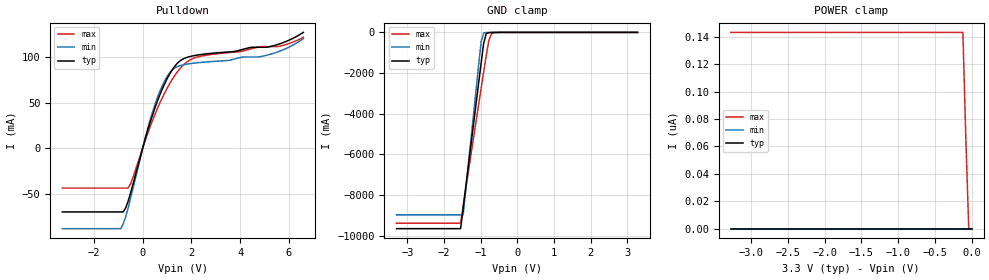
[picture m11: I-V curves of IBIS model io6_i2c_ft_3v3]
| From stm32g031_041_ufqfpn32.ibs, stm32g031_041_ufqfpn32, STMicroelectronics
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|   Model io6_i2c_ft_3v3
[Model]  io6_i2c_ft_3v3
Model_type I/O_open_drain
Polarity   Non-Inverting
Enable   Active-High
Vinl =   0.990000V
Vinh =   2.310000V
Vmeas =  1.650000V
Cref =   30.000000pF
Rref =   100.000000
Vref =   3.600000V
C_comp   2.033100pF   1.980600pF   2.082100pF
[Temperature Range]   25.000000   -40.000000   0.125000k
[Pullup Reference]   3.300000V   3.000000V   3.600000V
[Pulldown Reference]   0.0V   0.0V   0.0V
[POWER Clamp Reference]   3.300000V   3.000000V   3.600000V
[GND Clamp Reference]   0.0V   0.0V   0.0V
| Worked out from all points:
|   slope of the pulldown table from 0 to 0.495 V, typ, clamps not added: 11.3 ohm
|   GND clamp passes 1 mA (typ) near -0.58 V on its own axis
[Pulldown]
|Voltage   I(typ)   I(min)   I(max)
-3.3V     -70.17mA   -88.58mA   -43.95mA
-900mV    -70.17mA   -88.58mA   -43.95mA
-700mV    -65.85mA   -75.74mA   -43.95mA
-500mV    -49.6mA    -55.5mA    -39.37mA
100mV     9.759mA    10.83mA    8.012mA
500mV     44.06mA    47.69mA    36.87mA
900mV     70.75mA    73.99mA    60.62mA
1.3V      89.49mA    87.96mA    79.19mA
1.7V      98.65mA    91.88mA    92.3mA
2.2V      102.2mA    93.84mA    99.89mA
5V        111.1mA    101.7mA    111.8mA
6.6V      127.4mA    120.5mA    122mA
[GND_clamp]
|Voltage   I(typ)   I(min)   I(max)
-3.3V     -9.654A    -8.974A    -9.386A
-1.55V    -9.654A    -8.974A    -9.386A
-1.48V    -8.632A    -8.974A    -8.549A
-990mV    -1.519A    -464.6mA   -2.752A
-920mV    -535.3mA   -33.4mA    -1.941A
-850mV    -61.84mA   -8.927mA   -1.147A
-780mV    -11.5mA    -4.931mA   -400.9mA
-710mV    -4.633mA   -2.361mA   -72.05mA
-640mV    -2.18mA    -760.8uA   -15.81mA
3.28V     0A         0A         0A
[POWER_clamp]
|Voltage   I(typ)   I(min)   I(max)
-3.28V    0A         0A         143.3nA
-120mV    0A         0A         143.3nA
-80mV     0A         0A         66.35nA
-40mV     0A         0A         0A
0V        0A         0A         0A
[Ramp]
| variable   typ   min   max
dV/dt_r  1.60433/0.70922n   1.48592/0.61239n   1.67459/0.71435n
dV/dt_f  1.60433/1.86350n   1.48592/1.89955n   1.67459/2.07939n
R_load = 50.000000
|End [Model] io6_i2c_ft_3v3
